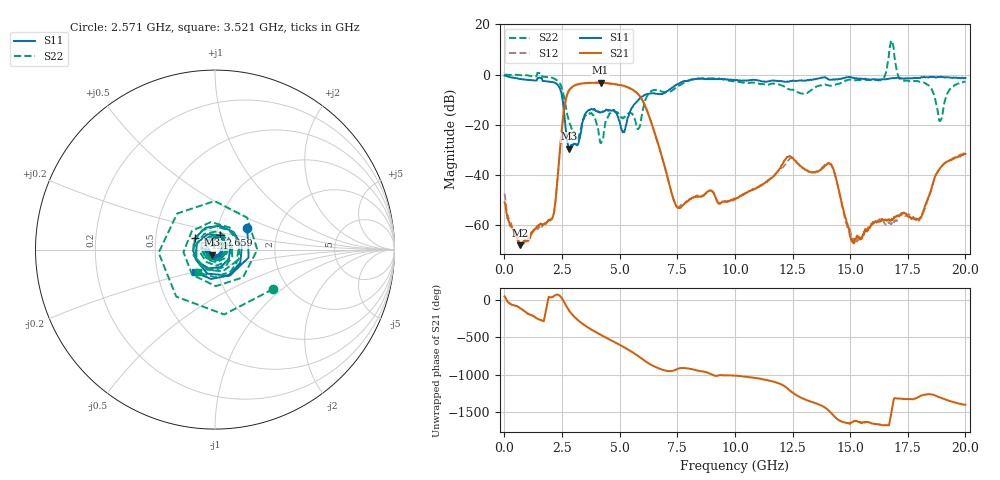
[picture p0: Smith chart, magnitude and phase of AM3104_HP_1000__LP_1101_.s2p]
!Created with skrf (http://scikit-rf.org).
# Hz S RI R 50.0
!freq ReS11 ImS11 ReS21 ImS21 ReS12 ImS12 ReS22 ImS22
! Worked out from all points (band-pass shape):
!   1601 points, 10 MHz to 20 GHz, reference 50 ohm
!   highest |S21| = -3.18 dB at 4.17 GHz (marker M1); lowest = -68.2 dB at 684.7 MHz (marker M2)
!   |S21| within 3 dB of the highest: 2.814 GHz to 5.59 GHz (2.776 GHz wide, 66.1 % of centre)
!   lowest |S11| = -29.6 dB at 2.809 GHz (marker M3), VSWR 1.07, Z = 48.3 - j2.76 ohm
!   |S11| at or under -10 dB: 2.525 GHz to 5.818 GHz (3.292 GHz wide, 78.9 % of centre)
!   |S22| runs from -27.3 to 13.6 dB; largest |S21 - S12| = 0.07
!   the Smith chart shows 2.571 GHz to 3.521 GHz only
!   S11 on the Smith chart (normalised r, x): 2.571 GHz: 1.39, +0.36; 2.659 GHz: 1.05, +0.17; 3.421 GHz: 0.80, +0.11; 3.521 GHz: 0.78, -0.20
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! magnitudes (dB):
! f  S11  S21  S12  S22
! 10 MHz  -0.4  -51.0  -47.4  0.0
! 684.7 MHz  -1.8  -68.2  -68.0  -0.2
! 2.084 GHz  -3.0  -57.3  -57.1  -1.3
! 2.571 GHz  -13.2  -15.3  -15.3  -8.2
! 2.659 GHz  -21.4  -10.2  -10.2  -12.5
! 2.809 GHz  -29.6  -6.2  -6.3  -18.8
! 3.346 GHz  -21.4  -3.6  -3.6  -20.6
! 3.421 GHz  -17.8  -3.5  -3.5  -17.9
! 3.521 GHz  -15.5  -3.4  -3.5  -16.1
! 4.17 GHz  -15.1  -3.2  -3.2  -27.3
! 5.157 GHz  -22.8  -4.4  -4.5  -17.4
! 5.795 GHz  -10.3  -7.7  -7.8  -21.8
! 6.682 GHz  -7.8  -28.0  -28.0  -6.3
! 7.531 GHz  -3.7  -53.2  -52.8  -4.7
! 10.01 GHz  -2.3  -49.7  -49.8  -2.9
! 13.34 GHz  -2.2  -39.1  -39.1  -6.0
! 14.2 GHz  -2.1  -36.3  -36.6  -4.4
! 15.09 GHz  -1.2  -66.4  -64.1  -2.2
! 16.68 GHz  -1.6  -58.1  -59.2  7.3
! 18.03 GHz  -1.4  -57.5  -57.3  -2.9
! 18.91 GHz  -0.8  -37.2  -37.2  -18.4
! 20 GHz  -1.3  -31.6  -31.1  -2.8
